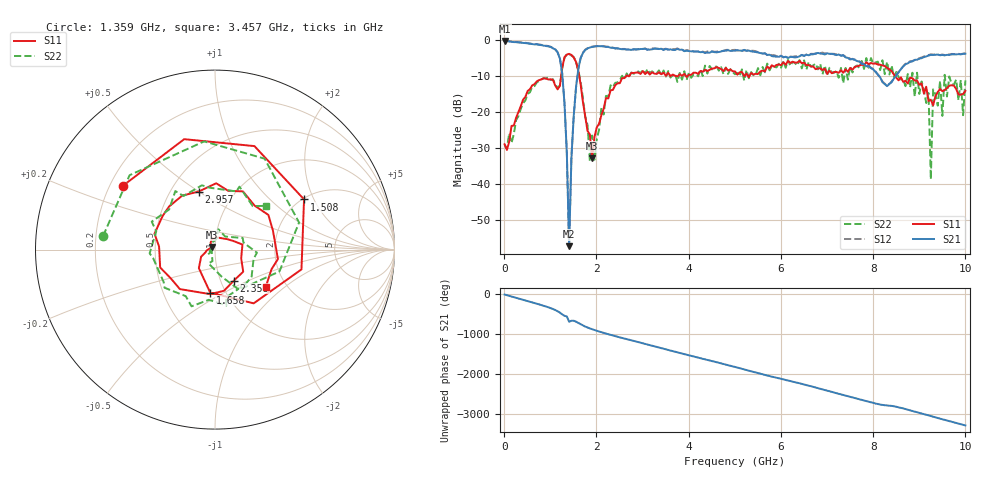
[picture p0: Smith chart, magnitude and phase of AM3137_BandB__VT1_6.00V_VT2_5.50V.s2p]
! Date/Time: Tue, Nov 13, 2018 4:52 PM
! Network Analyzer: Agilent Technologies E8364B Rev: A.07.50.67
! Sweep from 0.010 to 10.000 GHz, 201 Points, Sweep Type: LIN
! Power Supply: 6.001 V, 0.002 A
# Hz S DB R 50
!freq MagS11 AngS11 MagS21 AngS21 MagS12 AngS12 MagS22 AngS22
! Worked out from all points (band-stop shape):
!   201 points, 10 MHz to 10 GHz, reference 50 ohm
!   highest |S21| = -0.31 dB at 10 MHz (marker M1); lowest = -57.2 dB at 1.409 GHz (marker M2)
!   |S21| within 3 dB of the highest: start of sweep to 1.147 GHz; 1.728 GHz to 4.22 GHz (2.492 GHz wide, 83.8 % of centre)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
!   lowest |S11| = -32.8 dB at 1.908 GHz (marker M3), VSWR 1.05, Z = 48.2 + j1.41 ohm
!   |S11| at or under -10 dB: start of sweep to 1.236 GHz; 1.627 GHz to 2.648 GHz (1.022 GHz wide, 47.8 % of centre); 8.471 GHz to end of sweep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
!   |S22| runs from -38.7 to -4.0 dB; largest |S21 - S12| = 0.032
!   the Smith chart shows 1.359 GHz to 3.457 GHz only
!   S11 on the Smith chart (normalised r, x): 1.359 GHz: 0.25, +0.29; 1.508 GHz: 2.03, +1.68; 1.658 GHz: 0.85, -0.43; 2.358 GHz: 1.16, -0.42; 2.957 GHz: 0.68, +0.50; 3.457 GHz: 1.57, -0.74
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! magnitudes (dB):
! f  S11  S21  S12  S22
! 10 MHz  -28.9  -0.3  -0.2  -29.1
! 1.159 GHz  -13.7  -3.5  -3.4  -13.3
! 1.359 GHz  -4.1  -31.2  -31.2  -4.0
! 1.409 GHz  -3.9  -57.2  -56.9  -4.0
! 1.508 GHz  -4.9  -21.1  -21.0  -4.8
! 1.658 GHz  -12.3  -5.1  -5.0  -11.7
! 1.708 GHz  -17.3  -3.6  -3.5  -16.2
! 1.858 GHz  -26.2  -2.2  -2.0  -33.7
! 1.908 GHz  -32.8  -2.0  -1.9  -26.5
! 2.358 GHz  -13.9  -2.2  -2.2  -13.1
! 2.957 GHz  -9.5  -2.6  -2.5  -9.3
! 3.357 GHz  -9.0  -2.6  -2.5  -8.5
! 3.457 GHz  -9.1  -2.8  -2.6  -8.5
! 5.005 GHz  -8.8  -3.0  -2.8  -9.5
! 6.703 GHz  -7.4  -4.0  -3.9  -7.1
! 8.352 GHz  -8.2  -12.2  -12.2  -9.6
! 9.201 GHz  -17.0  -4.3  -4.2  -14.7
! 9.251 GHz  -16.6  -4.2  -4.0  -38.7
! 9.301 GHz  -18.2  -4.2  -4.1  -13.7
! 9.9 GHz  -15.2  -4.0  -4.0  -11.1
! 9.95 GHz  -15.0  -3.9  -3.8  -20.9
! 10 GHz  -14.2  -3.9  -3.8  -11.3
